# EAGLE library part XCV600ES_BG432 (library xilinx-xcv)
xcv600es_bg432 edit this description Auto generated by make-symbol-device-package-bsdl.ulp Rev. 26 Source: xcv600es_bg432.bsd
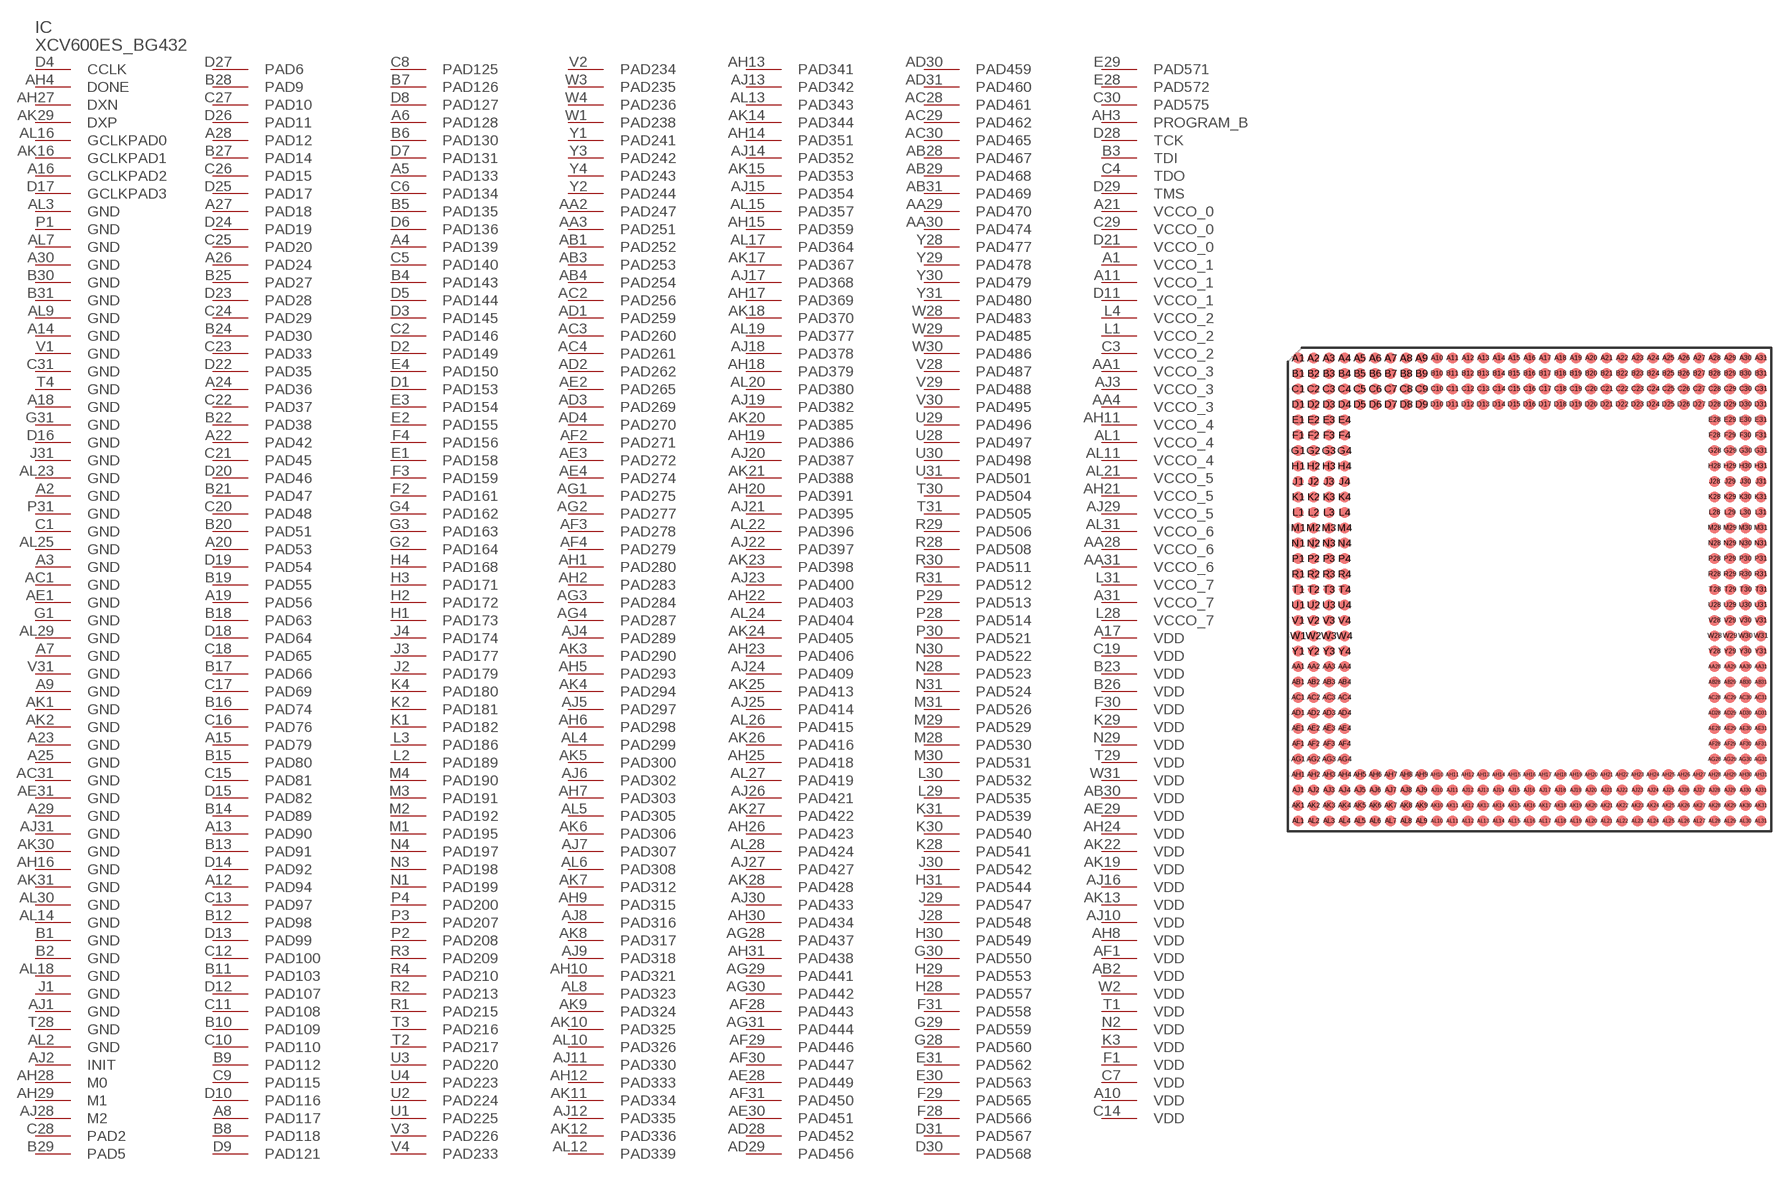
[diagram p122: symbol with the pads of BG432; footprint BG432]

Designator prefix IC

## XCV600ES_BG432 (OC_FARNELL: unknown; OC_NEWARK: unknown)  [BG432]
A1  VCCO_1  pwr
A2  GND  pwr
A3  GND  pwr
A4  PAD139
A5  PAD133
A6  PAD128
A7  GND  pwr
A8  PAD117
A9  GND  pwr
A10  VDD  pwr
A11  VCCO_1  pwr
A12  PAD94
A13  PAD90
A14  GND  pwr
A15  PAD79
A16  GCLKPAD2  in
A17  VDD  pwr
A18  GND  pwr
A19  PAD56
A20  PAD53
A21  VCCO_0  pwr
A22  PAD42
A23  GND  pwr
A24  PAD36
A25  GND  pwr
A26  PAD24
A27  PAD18
A28  PAD12
A29  GND  pwr
A30  GND  pwr
A31  VCCO_7  pwr
AA1  VCCO_3  pwr
AA2  PAD247
AA3  PAD251
AA4  VCCO_3  pwr
AA28  VCCO_6  pwr
AA29  PAD470
AA30  PAD474
AA31  VCCO_6  pwr
AB1  PAD252
AB2  VDD  pwr
AB3  PAD253
AB4  PAD254
AB28  PAD467
AB29  PAD468
AB30  VDD  pwr
AB31  PAD469
AC1  GND  pwr
AC2  PAD256
AC3  PAD260
AC4  PAD261
AC28  PAD461
AC29  PAD462
AC30  PAD465
AC31  GND  pwr
AD1  PAD259
AD2  PAD262
AD3  PAD269
AD4  PAD270
AD28  PAD452
AD29  PAD456
AD30  PAD459
AD31  PAD460
AE1  GND  pwr
AE2  PAD265
AE3  PAD272
AE4  PAD274
AE28  PAD449
AE29  VDD  pwr
AE30  PAD451
AE31  GND  pwr
AF1  VDD  pwr
AF2  PAD271
AF3  PAD278
AF4  PAD279
AF28  PAD443
AF29  PAD446
AF30  PAD447
AF31  PAD450
AG1  PAD275
AG2  PAD277
AG3  PAD284
AG4  PAD287
AG28  PAD437
AG29  PAD441
AG30  PAD442
AG31  PAD444
AH1  PAD280
AH2  PAD283
AH3  PROGRAM_B  in
AH4  DONE
AH5  PAD293
AH6  PAD298
AH7  PAD303
AH8  VDD  pwr
AH9  PAD315
AH10  PAD321
AH11  VCCO_4  pwr
AH12  PAD333
AH13  PAD341
AH14  PAD351
AH15  PAD359
AH16  GND  pwr
AH17  PAD369
AH18  PAD379
AH19  PAD386
AH20  PAD391
AH21  VCCO_5  pwr
AH22  PAD403
AH23  PAD406
AH24  VDD  pwr
AH25  PAD418
AH26  PAD423
AH27  DXN  pas
AH28  M0  in
AH29  M1  in
AH30  PAD434
AH31  PAD438
AJ1  GND  pwr
AJ2  INIT
AJ3  VCCO_3  pwr
AJ4  PAD289
AJ5  PAD297
AJ6  PAD302
AJ7  PAD307
AJ8  PAD316
AJ9  PAD318
AJ10  VDD  pwr
AJ11  PAD330
AJ12  PAD335
AJ13  PAD342
AJ14  PAD352
AJ15  PAD354
AJ16  VDD  pwr
AJ17  PAD368
AJ18  PAD378
AJ19  PAD382
AJ20  PAD387
AJ21  PAD395
AJ22  PAD397
AJ23  PAD400
AJ24  PAD409
AJ25  PAD414
AJ26  PAD421
AJ27  PAD427
AJ28  M2  in
AJ29  VCCO_5  pwr
AJ30  PAD433
AJ31  GND  pwr
AK1  GND  pwr
AK2  GND  pwr
AK3  PAD290
AK4  PAD294
AK5  PAD300
AK6  PAD306
AK7  PAD312
AK8  PAD317
AK9  PAD324
AK10  PAD325
AK11  PAD334
AK12  PAD336
AK13  VDD  pwr
AK14  PAD344
AK15  PAD353
AK16  GCLKPAD1  in
AK17  PAD367
AK18  PAD370
AK19  VDD  pwr
AK20  PAD385
AK21  PAD388
AK22  VDD  pwr
AK23  PAD398
AK24  PAD405
AK25  PAD413
AK26  PAD416
AK27  PAD422
AK28  PAD428
AK29  DXP  pas
AK30  GND  pwr
AK31  GND  pwr
AL1  VCCO_4  pwr
AL2  GND  pwr
AL3  GND  pwr
AL4  PAD299
AL5  PAD305
AL6  PAD308
AL7  GND  pwr
AL8  PAD323
AL9  GND  pwr
AL10  PAD326
AL11  VCCO_4  pwr
AL12  PAD339
AL13  PAD343
AL14  GND  pwr
AL15  PAD357
AL16  GCLKPAD0  in
AL17  PAD364
AL18  GND  pwr
AL19  PAD377
AL20  PAD380
AL21  VCCO_5  pwr
AL22  PAD396
AL23  GND  pwr
AL24  PAD404
AL25  GND  pwr
AL26  PAD415
AL27  PAD419
AL28  PAD424
AL29  GND  pwr
AL30  GND  pwr
AL31  VCCO_6  pwr
B1  GND  pwr
B2  GND  pwr
B3  TDI  in
B4  PAD143
B5  PAD135
B6  PAD130
B7  PAD126
B8  PAD118
B9  PAD112
B10  PAD109
B11  PAD103
B12  PAD98
B13  PAD91
B14  PAD89
B15  PAD80
B16  PAD74
B17  PAD66
B18  PAD63
B19  PAD55
B20  PAD51
B21  PAD47
B22  PAD38
B23  VDD  pwr
B24  PAD30
B25  PAD27
B26  VDD  pwr
B27  PAD14
B28  PAD9
B29  PAD5
B30  GND  pwr
B31  GND  pwr
C1  GND  pwr
C2  PAD146
C3  VCCO_2  pwr
C4  TDO  out
C5  PAD140
C6  PAD134
C7  VDD  pwr
C8  PAD125
C9  PAD115
C10  PAD110
C11  PAD108
C12  PAD100
C13  PAD97
C14  VDD  pwr
C15  PAD81
C16  PAD76
C17  PAD69
C18  PAD65
C19  VDD  pwr
C20  PAD48
C21  PAD45
C22  PAD37
C23  PAD33
C24  PAD29
C25  PAD20
C26  PAD15
C27  PAD10
C28  PAD2
C29  VCCO_0  pwr
C30  PAD575
C31  GND  pwr
D1  PAD153
D2  PAD149
D3  PAD145
D4  CCLK
D5  PAD144
D6  PAD136
D7  PAD131
D8  PAD127
D9  PAD121
D10  PAD116
D11  VCCO_1  pwr
D12  PAD107
D13  PAD99
D14  PAD92
D15  PAD82
D16  GND  pwr
D17  GCLKPAD3  in
D18  PAD64
D19  PAD54
D20  PAD46
D21  VCCO_0  pwr
D22  PAD35
D23  PAD28
D24  PAD19
D25  PAD17
D26  PAD11
D27  PAD6
D28  TCK  in
D29  TMS  in
D30  PAD568
D31  PAD567
E1  PAD158
E2  PAD155
E3  PAD154
E4  PAD150
E28  PAD572
E29  PAD571
E30  PAD563
E31  PAD562
F1  VDD  pwr
F2  PAD161
F3  PAD159
F4  PAD156
F28  PAD566
F29  PAD565
F30  VDD  pwr
F31  PAD558
G1  GND  pwr
G2  PAD164
G3  PAD163
G4  PAD162
G28  PAD560
G29  PAD559
G30  PAD550
G31  GND  pwr
H1  PAD173
H2  PAD172
H3  PAD171
H4  PAD168
H28  PAD557
H29  PAD553
H30  PAD549
H31  PAD544
J1  GND  pwr
J2  PAD179
J3  PAD177
J4  PAD174
J28  PAD548
J29  PAD547
J30  PAD542
J31  GND  pwr
K1  PAD182
K2  PAD181
K3  VDD  pwr
K4  PAD180
K28  PAD541
K29  VDD  pwr
K30  PAD540
K31  PAD539
L1  VCCO_2  pwr
L2  PAD189
L3  PAD186
L4  VCCO_2  pwr
L28  VCCO_7  pwr
L29  PAD535
L30  PAD532
L31  VCCO_7  pwr
M1  PAD195
M2  PAD192
M3  PAD191
M4  PAD190
M28  PAD530
M29  PAD529
M30  PAD531
M31  PAD526
N1  PAD199
N2  VDD  pwr
N3  PAD198
N4  PAD197
N28  PAD523
N29  VDD  pwr
N30  PAD522
N31  PAD524
P1  GND  pwr
P2  PAD208
P3  PAD207
P4  PAD200
P28  PAD514
P29  PAD513
P30  PAD521
P31  GND  pwr
R1  PAD215
R2  PAD213
R3  PAD209
R4  PAD210
R28  PAD508
R29  PAD506
R30  PAD511
R31  PAD512
T1  VDD  pwr
T2  PAD217
T3  PAD216
T4  GND  pwr
T28  GND  pwr
T29  VDD  pwr
T30  PAD504
T31  PAD505
U1  PAD225
U2  PAD224
U3  PAD220
U4  PAD223
U28  PAD497
U29  PAD496
U30  PAD498
U31  PAD501
V1  GND  pwr
V2  PAD234
V3  PAD226
V4  PAD233
V28  PAD487
V29  PAD488
V30  PAD495
V31  GND  pwr
W1  PAD238
W2  VDD  pwr
W3  PAD235
W4  PAD236
W28  PAD483
W29  PAD485
W30  PAD486
W31  VDD  pwr
Y1  PAD241
Y2  PAD244
Y3  PAD242
Y4  PAD243
Y28  PAD477
Y29  PAD478
Y30  PAD479
Y31  PAD480

## Footprint BG432 (pad centres in mm)
xcv300_bg432 edit this description Auto generated by make-symbol-device-package-bsdl.ulp Rev. 26 Source: xcv300_bg432.bsd
smd 0.9 x 0.9: A1 -19.05,19.05; A2 -17.78,19.05; A3 -16.51,19.05; A4 -15.24,19.05; A5 -13.97,19.05; A6 -12.7,19.05; A7 -11.43,19.05; A8 -10.16,19.05; A9 -8.89,19.05; A10 -7.62,19.05; A11 -6.35,19.05; A12 -5.08,19.05; A13 -3.81,19.05; A14 -2.54,19.05; A15 -1.27,19.05; A16 0,19.05; A17 1.27,19.05; A18 2.54,19.05; A19 3.81,19.05; A20 5.08,19.05; A21 6.35,19.05; A22 7.62,19.05; A23 8.89,19.05; A24 10.16,19.05; A25 11.43,19.05; A26 12.7,19.05; A27 13.97,19.05; A28 15.24,19.05; A29 16.51,19.05; A30 17.78,19.05; A31 19.05,19.05; AA1 -19.05,-6.35; AA2 -17.78,-6.35; AA3 -16.51,-6.35; AA4 -15.24,-6.35; AA28 15.24,-6.35; AA29 16.51,-6.35; AA30 17.78,-6.35; AA31 19.05,-6.35; AB1 -19.05,-7.62; AB2 -17.78,-7.62; AB3 -16.51,-7.62; AB4 -15.24,-7.62; AB28 15.24,-7.62; AB29 16.51,-7.62; AB30 17.78,-7.62; AB31 19.05,-7.62; AC1 -19.05,-8.89; AC2 -17.78,-8.89; AC3 -16.51,-8.89; AC4 -15.24,-8.89; AC28 15.24,-8.89; AC29 16.51,-8.89; AC30 17.78,-8.89; AC31 19.05,-8.89; AD1 -19.05,-10.16; AD2 -17.78,-10.16; AD3 -16.51,-10.16; AD4 -15.24,-10.16; AD28 15.24,-10.16; AD29 16.51,-10.16; AD30 17.78,-10.16; AD31 19.05,-10.16; AE1 -19.05,-11.43; AE2 -17.78,-11.43; AE3 -16.51,-11.43; AE4 -15.24,-11.43; AE28 15.24,-11.43; AE29 16.51,-11.43; AE30 17.78,-11.43; AE31 19.05,-11.43; AF1 -19.05,-12.7; AF2 -17.78,-12.7; AF3 -16.51,-12.7; AF4 -15.24,-12.7; AF28 15.24,-12.7; AF29 16.51,-12.7; AF30 17.78,-12.7; AF31 19.05,-12.7; AG1 -19.05,-13.97; AG2 -17.78,-13.97; AG3 -16.51,-13.97; AG4 -15.24,-13.97; AG28 15.24,-13.97; AG29 16.51,-13.97; AG30 17.78,-13.97; AG31 19.05,-13.97; AH1 -19.05,-15.24; AH2 -17.78,-15.24; AH3 -16.51,-15.24; AH4 -15.24,-15.24; AH5 -13.97,-15.24; AH6 -12.7,-15.24; AH7 -11.43,-15.24; AH8 -10.16,-15.24; AH9 -8.89,-15.24; AH10 -7.62,-15.24; AH11 -6.35,-15.24; AH12 -5.08,-15.24; AH13 -3.81,-15.24; AH14 -2.54,-15.24; AH15 -1.27,-15.24; AH16 0,-15.24; AH17 1.27,-15.24; AH18 2.54,-15.24; AH19 3.81,-15.24; AH20 5.08,-15.24; AH21 6.35,-15.24; AH22 7.62,-15.24; AH23 8.89,-15.24; AH24 10.16,-15.24; AH25 11.43,-15.24; AH26 12.7,-15.24; AH27 13.97,-15.24; AH28 15.24,-15.24; AH29 16.51,-15.24; AH30 17.78,-15.24; AH31 19.05,-15.24; AJ1 -19.05,-16.51; AJ2 -17.78,-16.51; AJ3 -16.51,-16.51; AJ4 -15.24,-16.51; AJ5 -13.97,-16.51; AJ6 -12.7,-16.51; AJ7 -11.43,-16.51; AJ8 -10.16,-16.51; AJ9 -8.89,-16.51; AJ10 -7.62,-16.51; AJ11 -6.35,-16.51; AJ12 -5.08,-16.51; AJ13 -3.81,-16.51; AJ14 -2.54,-16.51; AJ15 -1.27,-16.51; AJ16 0,-16.51; AJ17 1.27,-16.51; AJ18 2.54,-16.51; AJ19 3.81,-16.51; AJ20 5.08,-16.51; AJ21 6.35,-16.51; AJ22 7.62,-16.51; AJ23 8.89,-16.51; AJ24 10.16,-16.51; AJ25 11.43,-16.51; AJ26 12.7,-16.51; AJ27 13.97,-16.51; AJ28 15.24,-16.51; AJ29 16.51,-16.51; AJ30 17.78,-16.51; AJ31 19.05,-16.51; AK1 -19.05,-17.78; AK2 -17.78,-17.78; AK3 -16.51,-17.78; AK4 -15.24,-17.78; AK5 -13.97,-17.78; AK6 -12.7,-17.78; AK7 -11.43,-17.78; AK8 -10.16,-17.78; AK9 -8.89,-17.78; AK10 -7.62,-17.78; AK11 -6.35,-17.78; AK12 -5.08,-17.78; AK13 -3.81,-17.78; AK14 -2.54,-17.78; AK15 -1.27,-17.78; AK16 0,-17.78; AK17 1.27,-17.78; AK18 2.54,-17.78; AK19 3.81,-17.78; AK20 5.08,-17.78; AK21 6.35,-17.78; AK22 7.62,-17.78; AK23 8.89,-17.78; AK24 10.16,-17.78; AK25 11.43,-17.78; AK26 12.7,-17.78; AK27 13.97,-17.78; AK28 15.24,-17.78; AK29 16.51,-17.78; AK30 17.78,-17.78; AK31 19.05,-17.78; AL1 -19.05,-19.05; AL2 -17.78,-19.05; AL3 -16.51,-19.05; AL4 -15.24,-19.05; AL5 -13.97,-19.05; AL6 -12.7,-19.05; AL7 -11.43,-19.05; AL8 -10.16,-19.05; AL9 -8.89,-19.05; AL10 -7.62,-19.05; AL11 -6.35,-19.05; AL12 -5.08,-19.05; AL13 -3.81,-19.05; AL14 -2.54,-19.05; AL15 -1.27,-19.05; AL16 0,-19.05; AL17 1.27,-19.05; AL18 2.54,-19.05; AL19 3.81,-19.05; AL20 5.08,-19.05; AL21 6.35,-19.05; AL22 7.62,-19.05; AL23 8.89,-19.05; AL24 10.16,-19.05; AL25 11.43,-19.05; AL26 12.7,-19.05; AL27 13.97,-19.05; AL28 15.24,-19.05; AL29 16.51,-19.05; AL30 17.78,-19.05; AL31 19.05,-19.05; B1 -19.05,17.78; B2 -17.78,17.78; B3 -16.51,17.78; B4 -15.24,17.78; B5 -13.97,17.78; B6 -12.7,17.78; B7 -11.43,17.78; B8 -10.16,17.78; B9 -8.89,17.78; B10 -7.62,17.78; B11 -6.35,17.78; B12 -5.08,17.78; B13 -3.81,17.78; B14 -2.54,17.78; B15 -1.27,17.78; B16 0,17.78; B17 1.27,17.78; B18 2.54,17.78; B19 3.81,17.78; B20 5.08,17.78; B21 6.35,17.78; B22 7.62,17.78; B23 8.89,17.78; B24 10.16,17.78; B25 11.43,17.78; B26 12.7,17.78; B27 13.97,17.78; B28 15.24,17.78; B29 16.51,17.78; B30 17.78,17.78; B31 19.05,17.78; C1 -19.05,16.51; C2 -17.78,16.51; C3 -16.51,16.51; C4 -15.24,16.51; C5 -13.97,16.51; C6 -12.7,16.51; C7 -11.43,16.51; C8 -10.16,16.51; C9 -8.89,16.51; C10 -7.62,16.51; C11 -6.35,16.51; C12 -5.08,16.51; C13 -3.81,16.51; C14 -2.54,16.51; C15 -1.27,16.51; C16 0,16.51; C17 1.27,16.51; C18 2.54,16.51; C19 3.81,16.51; C20 5.08,16.51; C21 6.35,16.51; C22 7.62,16.51; C23 8.89,16.51; C24 10.16,16.51; C25 11.43,16.51; C26 12.7,16.51; C27 13.97,16.51; C28 15.24,16.51; C29 16.51,16.51; C30 17.78,16.51; C31 19.05,16.51; D1 -19.05,15.24; D2 -17.78,15.24; D3 -16.51,15.24; D4 -15.24,15.24; D5 -13.97,15.24; D6 -12.7,15.24; D7 -11.43,15.24; D8 -10.16,15.24; D9 -8.89,15.24; D10 -7.62,15.24; D11 -6.35,15.24; D12 -5.08,15.24; D13 -3.81,15.24; D14 -2.54,15.24; D15 -1.27,15.24; D16 0,15.24; D17 1.27,15.24; D18 2.54,15.24; D19 3.81,15.24; D20 5.08,15.24; D21 6.35,15.24; D22 7.62,15.24; D23 8.89,15.24; D24 10.16,15.24; D25 11.43,15.24; D26 12.7,15.24; D27 13.97,15.24; D28 15.24,15.24; D29 16.51,15.24; D30 17.78,15.24; D31 19.05,15.24; E1 -19.05,13.97; E2 -17.78,13.97; E3 -16.51,13.97; E4 -15.24,13.97; E28 15.24,13.97; E29 16.51,13.97; E30 17.78,13.97; E31 19.05,13.97; F1 -19.05,12.7; F2 -17.78,12.7; F3 -16.51,12.7; F4 -15.24,12.7; F28 15.24,12.7; F29 16.51,12.7; F30 17.78,12.7; F31 19.05,12.7; G1 -19.05,11.43; G2 -17.78,11.43; G3 -16.51,11.43; G4 -15.24,11.43; G28 15.24,11.43; G29 16.51,11.43; G30 17.78,11.43; G31 19.05,11.43; H1 -19.05,10.16; H2 -17.78,10.16; H3 -16.51,10.16; H4 -15.24,10.16; H28 15.24,10.16; H29 16.51,10.16; H30 17.78,10.16; H31 19.05,10.16; J1 -19.05,8.89; J2 -17.78,8.89; J3 -16.51,8.89; J4 -15.24,8.89; J28 15.24,8.89; J29 16.51,8.89; J30 17.78,8.89; J31 19.05,8.89; K1 -19.05,7.62; K2 -17.78,7.62; K3 -16.51,7.62; K4 -15.24,7.62; K28 15.24,7.62; K29 16.51,7.62; K30 17.78,7.62; K31 19.05,7.62; L1 -19.05,6.35; L2 -17.78,6.35; L3 -16.51,6.35; L4 -15.24,6.35; L28 15.24,6.35; L29 16.51,6.35; L30 17.78,6.35; L31 19.05,6.35; M1 -19.05,5.08; M2 -17.78,5.08; M3 -16.51,5.08; M4 -15.24,5.08; M28 15.24,5.08; M29 16.51,5.08; M30 17.78,5.08; M31 19.05,5.08; N1 -19.05,3.81; N2 -17.78,3.81; N3 -16.51,3.81; N4 -15.24,3.81; N28 15.24,3.81; N29 16.51,3.81; N30 17.78,3.81; N31 19.05,3.81; P1 -19.05,2.54; P2 -17.78,2.54; P3 -16.51,2.54; P4 -15.24,2.54; P28 15.24,2.54; P29 16.51,2.54; P30 17.78,2.54; P31 19.05,2.54; R1 -19.05,1.27; R2 -17.78,1.27; R3 -16.51,1.27; R4 -15.24,1.27; R28 15.24,1.27; R29 16.51,1.27; R30 17.78,1.27; R31 19.05,1.27; T1 -19.05,0; T2 -17.78,0; T3 -16.51,0; T4 -15.24,0; T28 15.24,0; T29 16.51,0; T30 17.78,0; T31 19.05,0; U1 -19.05,-1.27; U2 -17.78,-1.27; U3 -16.51,-1.27; U4 -15.24,-1.27; U28 15.24,-1.27; U29 16.51,-1.27; U30 17.78,-1.27; U31 19.05,-1.27; V1 -19.05,-2.54; V2 -17.78,-2.54; V3 -16.51,-2.54; V4 -15.24,-2.54; V28 15.24,-2.54; V29 16.51,-2.54; V30 17.78,-2.54; V31 19.05,-2.54; W1 -19.05,-3.81; W2 -17.78,-3.81; W3 -16.51,-3.81; W4 -15.24,-3.81; W28 15.24,-3.81; W29 16.51,-3.81; W30 17.78,-3.81; W31 19.05,-3.81; Y1 -19.05,-5.08; Y2 -17.78,-5.08; Y3 -16.51,-5.08; Y4 -15.24,-5.08; Y28 15.24,-5.08; Y29 16.51,-5.08; Y30 17.78,-5.08; Y31 19.05,-5.08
